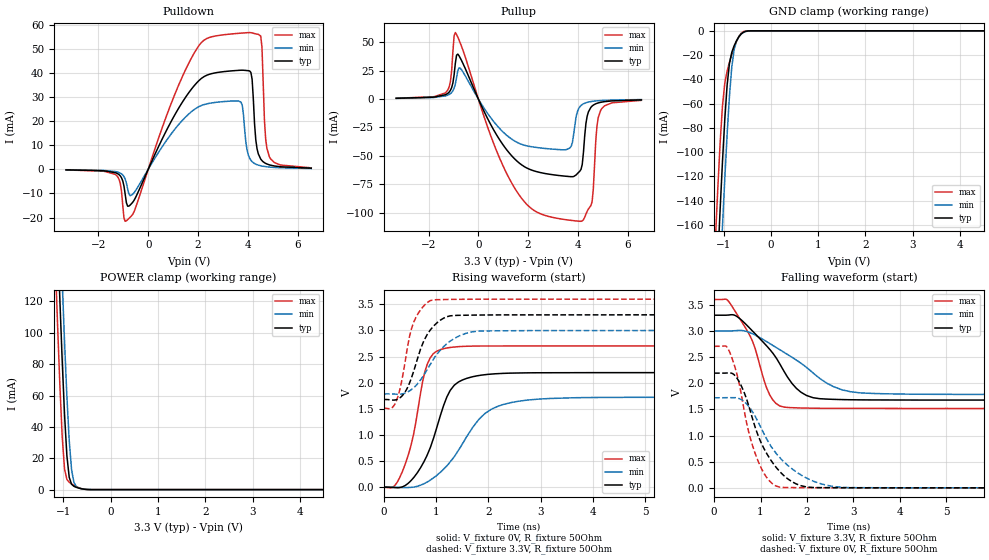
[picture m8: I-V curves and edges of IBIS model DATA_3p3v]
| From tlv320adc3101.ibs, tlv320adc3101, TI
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|   DATA_3p3v
[Model]   DATA_3p3v
Model_type   3-state
Polarity   Non-Inverting
Vmeas = 1.65
Vref = 0
Cref = 5pF
Rref = 1000000
|   typ   min   max
C_comp   1.339pF   1.297pF   1.403pF
[Voltage Range]   3.3   3   3.6
[Temperature Range]   27   85   -40
[Pullup Reference]   3.3   3   3.6
[Pulldown Reference]   -0   -0   -0
[Power Clamp Reference]   3.3   3   3.6
[GND Clamp Reference]   -0   -0   -0
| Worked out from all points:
|   slope of the pulldown table from 0 to 0.495 V, typ, clamps not added: 44.4 ohm
|   slope of the pullup table from 0 to 0.495 V, typ, clamps not added: 22.1 ohm
|   GND clamp passes 1 mA (typ) near -0.57 V on its own axis
|   POWER clamp passes 1 mA (typ) near -0.68 V on its own axis
|   falling waveform, V_fixture 3.3V, R_fixture 50Ohm: 20-80 % time 821ps typ, 1.18ns min, 534ps max; typ from 3.3 V to 1.68 V
|   rising waveform, V_fixture 0V, R_fixture 50Ohm: 20-80 % time 479ps typ, 758ps min, 333ps max; typ from 0 V to 2.19 V
|   rising waveform, V_fixture 3.3V, R_fixture 50Ohm: 20-80 % time 371ps typ, 535ps min, 263ps max; typ from 1.68 V to 3.3 V
|   falling waveform, V_fixture 0V, R_fixture 50Ohm: 20-80 % time 620ps typ, 828ps min, 440ps max; typ from 2.19 V to 0 V
[Pulldown]
|   Voltage   I(typ)   I(min)   I(max)
-3.3V     -212uA     -165.3uA   -254.7uA
-1.27V    -1.575mA   -1.029mA   -2.546mA
-874.5mV  -13.94mA   -5.795mA   -21.31mA
1.996V    36.36mA    25.76mA    50.68mA
3.729V    41.1mA     27.88mA    56.46mA
4.075V    40.76mA    4.602mA    56.7mA
4.175V    37.37mA    3.183mA    56.56mA
4.323V    12.16mA    2.143mA    56.16mA
4.521V    4.251mA    1.478mA    55.24mA
4.719V    2.467mA    1.123mA    12.61mA
4.867V    1.864mA    950.6uA    5.25mA
6.551V    483uA      342.8uA    619.6uA
[GND Clamp]
|   Voltage   I(typ)   I(min)   I(max)
-3.3V     -2.299A    -2.353A    -2.242A
-1.171V   -232.8mA   -290.6mA   -172mA
-1.122V   -189.5mA   -246.5mA   -130.6mA
-1.073V   -147.7mA   -203.4mA   -92.86mA
-1.023V   -108.3mA   -161.7mA   -62.19mA
-973.5mV  -72.99mA   -121.9mA   -43.14mA
-924mV    -44.7mA    -85.27mA   -33.16mA
-874.5mV  -26.76mA   -53.54mA   -25.94mA
-825mV    -17.66mA   -29.59mA   -19.51mA
-726mV    -8.242mA   -8.487mA   -8.64mA
-577.5mV  -1.101mA   -1.302mA   -631.4uA
6.551V    0A         0A         0A
[Pullup]
|   Voltage   I(typ)   I(min)   I(max)
-3.3V     578.4uA    489.8uA    654.2uA
-1.32V    3.711mA    2.67mA     5.332mA
-1.122V   7.569mA    4.654mA    15.35mA
-924mV    31.46mA    13.15mA    58.45mA
-726mV    36.01mA    27.07mA    49.17mA
1.551V    -54.69mA   -38.18mA   -81.66mA
3.63V     -68.27mA   -43.77mA   -106.6mA
4.075V    -63.64mA   -6.981mA   -107.7mA
4.571V    -6.28mA    -2.153mA   -90.59mA
4.769V    -3.834mA   -1.67mA    -23.47mA
4.917V    -2.95mA    -1.427mA   -9.967mA
6.551V    -815.7uA   -543.8uA   -1.215mA
[POWER Clamp]
|   Voltage   I(typ)   I(min)   I(max)
-3.3V     2.272A     2.321A     2.221A
-1.171V   206.1mA    260.3mA    148.4mA
-1.122V   162.9mA    216.6mA    106.1mA
-1.073V   121.3mA    174mA      66.87mA
-1.023V   82.27mA    132.9mA    33.78mA
-973.5mV  47.82mA    94.32mA    13.16mA
-924mV    21.64mA    59.55mA    6.5mA
-874.5mV  7.819mA    31.22mA    4.673mA
-825mV    3.429mA    12.77mA    3.618mA
-775.5mV  2.112mA    4.594mA    2.733mA
-726mV    1.457mA    1.977mA    1.951mA
6.551V    0A         0A         0A
[Ramp]
R_load = 50
|   typ   min   max
dV/dt_r   1.31544/4.79475e-010   1.03267/7.5778e-010   1.62416/3.32053e-010
dV/dt_f   0.973404/8.21409e-010  0.728771/1.18084e-009   1.24965/5.33814e-010
[Falling Waveform]
V_fixture = 3.3V
V_fixture_min = 3V
V_fixture_max = 3.6V
R_fixture = 50Ohm
C_fixture = 0F
|   Time   V(typ)   V(min)   V(max)
0s        3.3V       3V         3.6V
287ps     3.302V     3V         3.589V
653.7ps   3.154V     3V         3.091V
828.2ps   2.997V     2.944V     2.801V
1.195ns   2.65V      2.76V      1.782V
1.414ns   2.371V     2.641V     1.566V
1.677ns   1.997V     2.496V     1.533V
1.987ns   1.767V     2.304V     1.525V
2.937ns   1.684V     1.837V     1.519V
8.394ns   1.678V     1.785V     1.517V
[Rising Waveform]
V_fixture = 0V
V_fixture_min = 0V
V_fixture_max = 0V
R_fixture = 50Ohm
C_fixture = 0F
|   Time   V(typ)   V(min)   V(max)
0s        361.7uV    28.45uV    -1.17mV
184ps     -7.638mV   -353.6uV   8.999mV
347.1ps   3.15mV     -7.208mV   284.9mV
566.4ps   179.5mV    138.1uV    1.008V
784.5ps   524.8mV    74.22mV    2.214V
1.075ns   1.352V     280.2mV    2.63V
1.425ns   2.012V     704mV      2.69V
1.935ns   2.153V     1.411V     2.702V
2.435ns   2.183V     1.62V      2.703V
8.394ns   2.193V     1.721V     2.706V
[Rising Waveform]
V_fixture = 3.3V
V_fixture_min = 3V
V_fixture_max = 3.6V
R_fixture = 50Ohm
C_fixture = 0F
|   Time   V(typ)   V(min)   V(max)
0s        1.678V     1.785V     1.516V
222.1ps   1.671V     1.781V     1.617V
400ps     1.814V     1.799V     2.369V
489.1ps   1.992V     1.844V     2.883V
566.4ps   2.211V     1.9V       3.15V
764.5ps   2.803V     2.148V     3.471V
941.1ps   3.073V     2.437V     3.585V
1.346ns   3.287V     2.847V     3.596V
1.817ns   3.295V     2.987V     3.599V
8.394ns   3.3V       3V         3.6V
[Falling Waveform]
|Gnd
V_fixture = 0V
V_fixture_min = 0V
V_fixture_max = 0V
R_fixture = 50Ohm
C_fixture = 0F
|   Time   V(typ)   V(min)   V(max)
0s        2.193V     1.721V     2.706V
272.9ps   2.195V     1.723V     2.696V
485ps     2.107V     1.72V      2.197V
740.9ps   1.583V     1.563V     1.085V
884.7ps   1.159V     1.369V     658.1mV
1.128ns   666mV      943.1mV    204.9mV
1.331ns   399.2mV    665.9mV    36.37mV
1.869ns   41.87mV    248.9mV    3.726mV
2.582ns   3.416mV    25.24mV    1.506mV
8.394ns   -6.519uV   18.88uV    -5.148uV
